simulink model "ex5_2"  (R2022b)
settings: Solver=ode45  StartTime=0.0  StopTime=10.0  RelTol=1e-3  EnableMultiTasking=on

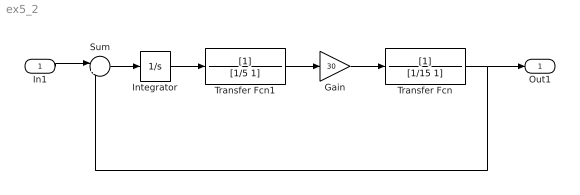
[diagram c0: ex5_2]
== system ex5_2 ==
  In1 : Inport
  Gain : Gain  Gain=30
  Integrator : Integrator
  Sum : Sum  Inputs=|+-
  Transfer Fcn : TransferFcn  Denominator=[1/15 1]
  Transfer Fcn1 : TransferFcn  Denominator=[1/5 1]
  Out1 : Outport
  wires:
  Transfer Fcn1/1 -> Gain/1
  Gain/1 -> Transfer Fcn/1
  Integrator/1 -> Transfer Fcn1/1
  In1/1 -> Sum/1
  Sum/1 -> Integrator/1
  Transfer Fcn/1 -> Sum/2, Out1/1
